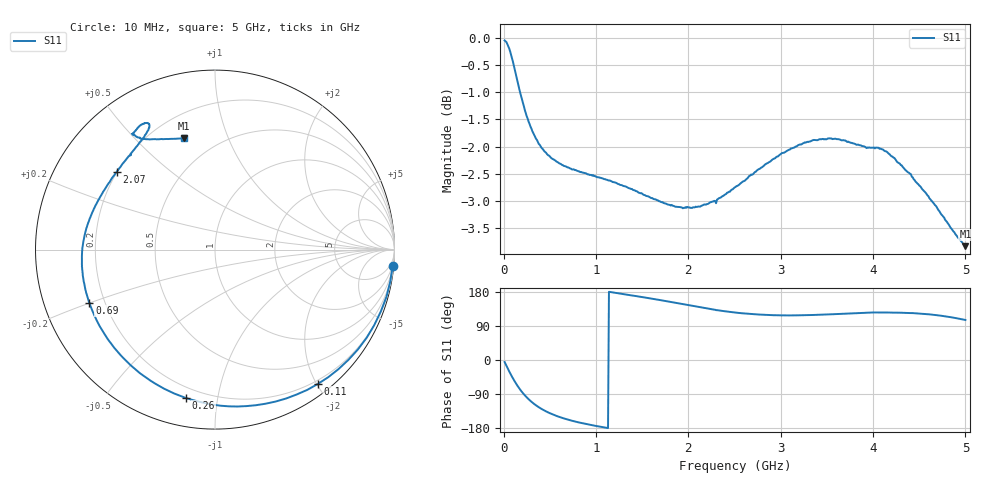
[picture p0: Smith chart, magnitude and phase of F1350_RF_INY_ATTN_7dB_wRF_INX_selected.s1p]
! S-parameters for RF_INY input IDT F1350 DPD Demodulator
! Date Measured:  2015-11-25  RGG
!  Port 1 = Pin 3 = RF_INY
! STATE: RF_INX selected, 7 dB attenuation (Gain = Gmax - 7 dB)
! RF Frequency:  10 MHz to 5000 MHz
! RF_INX, IF_I+, IF_I-, IF_Q+, and IF_Q- terminated
! 2300 MHz, 0 dBm signal applied to LO_IN
! Vcc = +5.00 Volts  Icc = approx 275 mA
! NOTES:  The device was measured on a custom printed circuit evaluation board with individual 50 ohm
!  microstrip lines to the RF and LO pins. The 50 ohm microstrip lines were de-embedded using reference
!  plane extensions
! Instrument Manufacturer:  Agilent Technologies
! Instrument Model:  E5071C
! Instrument Serial Number:  MY46419053
! Instrument Firmware Rev:  A.11.31
# HZ  S  RI R 50.00
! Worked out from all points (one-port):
!   500 points, 10 MHz to 5 GHz, reference 50 ohm
!   lowest |S11| = -3.8 dB at 5 GHz (marker M1), VSWR 4.61, Z = 16.6 + j35.2 ohm
!   |S11| at or under -10 dB: nowhere
!   S11 on the Smith chart (normalised r, x): 10 MHz: 1, -22; 110 MHz: 0.15, -2.01; 260 MHz: 0.14, -0.81; 690 MHz: 0.14, -0.20; 2.07 GHz: 0.20, +0.34; 5 GHz: 0.33, +0.70
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1e7  0.99 -0.0911
3e7  0.9552 -0.2629
5e7  0.8871 -0.4211
8e7  0.7438 -0.6138
1.1e8  0.5726 -0.7487
1.4e8  0.396 -0.8296
1.7e8  0.227 -0.8672
2.1e8  0.0317 -0.8698
2.6e8  -0.1625 -0.8267
3.3e8  -0.3575 -0.7314
4.1e8  -0.4998 -0.6146
5.1e8  -0.6067 -0.4839
6.4e8  -0.682 -0.3439
6.9e8  -0.6998 -0.2968
9.4e8  -0.7397 -0.112
1.26e9  -0.73 0.0608
1.57e9  -0.6843 0.2061
1.89e9  -0.603 0.354
2.07e9  -0.5469 0.4346
2.51e9  -0.4202 0.5958
2.82e9  -0.371 0.6669
3.13e9  -0.3695 0.7005
3.43e9  -0.3976 0.7021
3.76e9  -0.4342 0.6726
4.06e9  -0.4614 0.644
4.38e9  -0.4198 0.6241
4.69e9  -0.3309 0.6155
5e9  -0.1736 0.6196
